| IBIS file stm32f413_f423_wlcsp81.ibs
[IBIS ver] 4.2
[File name] stm32f413_f423_wlcsp81.ibs
[File Rev] 1.1
[Date]  18-05-2020
[Source] Data Created at STMicroelectronics
[Notes]  File originated from ELDO simulations. rev 1.1: removal of the rising/falling waveform I2C
[Disclaimer]  This information is for modeling purpose only and is
   not guaranted. The information is subject to change without
   notice.
[Copyright] Copyright 2020 STMicroelectronics Inc.
|   Component stm32f413_f423_wlcsp81
[Component] stm32f413_f423_wlcsp81
[Manufacturer] STMicroelectronics
[Package]
| variable   typ   min   max
R_pkg   0.0   0.0   0.0
L_pkg   0.0H   0.0H   0.0H
C_pkg   0.0F   0.0F   0.0F
[Pin]  signal_name   model_name   R_pin   L_pin   C_pin
A1 VDD_2_0 POWER
A2 PC10 io8p_arsudq_ft
A3 PA15 io8p_arsudq_ft
A4 PD0 io8p_arsudq_ft
A5 PB3 io8p_arsudq_i2c_ft
A6 PB5 io8p_ar3wsudq_ft
A7 BOOT0 vpp_test_hv
A8 VSS_3 GND
A9 VDD_3 POWER
B1 VSS_2_0 POWER
B2 PA14 io8p_arsudq_ft
B3 PA12 io8usb_lsfs_otg_ft
B4 PC12 io8p_arsudq_ft
B5 PB4 io8p_arsudq_i2cin_ft
B6 PB6 io8p_arsudq_i2cin_ft
B7 PB7 io8p_arsudq_i2cin_ft
B8 VSS GND
B9 VBAT POWER
C1 VCAP2_0 POWER
C2 PA13 io8p_arsudq_ft
C3 PA11 io8usb_lsfs_otg_ft
C4 PC11 io8p_arsudq_ft
C5 PD2 io8p_arsudq_ft
C6 PB8 io8p_arsudq_i2cin_ft
C7 PC1 io8p_arwsudq_ft_v33
C8 PC13-ANTI_TAMP io8p_arwsudq_ft_v33
C9 PC14-OSC32_IN io8p_arwsudq_ft
D1 PA10 io8usb_id_otg_ft
D2 PA9 io8usb_vbus_otg_ft
D3 PA8 io8p_arsudq_i2cin_ft
D4 PC7 io8p_arsudq_i2c_ft
D5 PC6 io8p_arsudq_i2c_ft
D6 PB9 io8p_arsudq_i2cin_ft
D7 PC2 io8p_arwsudq_ft
D8 VSS_5 GND
D9 PC15-OSC32_OUT io8p_arsudq_ft
E1 PC8 io8p_arsudq_ft
E2 PC9 io8p_arsudq_i2cin_ft
E3 PB14 io8p_arsudq_i2c_ft
E4 PB0 io8p_ar3wsudq_ft
E5 PA4 io8p_ar3wsudq_ft
E6 PA3 io8p_arwsudq_ft
E7 PC3 io8p_arwsudq_ft
E8 VDD_5 POWER
E9 PH0-OSC_IN io8p_arsudq_ft
F1 VDD_2_USB33 POWER
F2 PD9 io8p_arsudq_ft
F3 PB12 io8p_arsudq_ft
F4 PE13 io8p_arsudq_ft
F5 PA6 io8p_ar3wsudq_ft
F6 VSS GND
F7 VDDA POWER
F8 PC0 io8p_arwsudq_ft_v33
F9 PH1-OSC_OUT io8p_arsudq_ft
G1 PD10 io8p_arsudq_ft
G2 PB13 io8p_arsudq_ft
G3 PE14 io8p_arsudq_ft
G4 PE10 io8p_arsudq_ft
G5 PB1 io8p_ar3wsudq_ft
G6 PA5 io8p_ar3wsudq_ft
G7 PA0-WKUP io8p_arwsudq_ft_v33
G8 VREF+ POWER
G9 NRST ioreset_ft_v33
H1 PB15 io8p_arsudq_i2c_ft
H2 VCAP1_0 POWER
H3 PB10 io8p_arsudq_i2c_ft
H4 PE11 io8p_arsudq_ft
H5 PB2 io8p_arwsudq_ft
H6 PC4 io8p_arwsudq_ft
H7 VSS_4 GND
H8 PA1 io8p_arwsudq_ft
H9 VSSA GND
J1 VDD_1_0 POWER
J2 VSS_1_0 GND
J3 PE15 io8p_ar3wsudq_ft
J4 PE12 io8p_arsudq_ft
J5 PE9 io8p_arsudq_ft
J6 PC5 io8p_arwsudq_ft
J7 PA7 io8p_arwsudq_ft
J8 VDD_4 POWER
J9 PA2 io8p_arwsudq_ft
[Model Selector] io8p_ar3wsudq_ft
io8p00_ar3wsudq_ft_pd_lv  "SPEED00 1P8V, PD=40kOhm"
io8p00_ar3wsudq_ft_pu_lv  "SPEED00 1P8V, PU=40kOhm"
io8p00_ar3wsudq_ft_lv  "SPEED00 1P8V"
io8p01_ar3wsudq_ft_pd_lv  "SPEED01 1P8V, PD=40kOhm"
io8p01_ar3wsudq_ft_pu_lv  "SPEED01 1P8V, PU=40kOhm"
io8p01_ar3wsudq_ft_lv  "SPEED01 1P8V"
io8p10_ar3wsudq_ft_pd_lv  "SPEED10 1P8V, PD=40kOhm"
io8p10_ar3wsudq_ft_pu_lv  "SPEED10 1P8V, PU=40kOhm"
io8p10_ar3wsudq_ft_lv  "SPEED10 1P8V"
io8p11_ar3wsudq_ft_pd_lv  "SPEED11 1P8V, PD=40kOhm"
io8p11_ar3wsudq_ft_pu_lv  "SPEED11 1P8V, PU=40kOhm"
io8p11_ar3wsudq_ft_lv  "SPEED11 1P8V"
io8p00_ar3wsudq_ft_pd  "SPEED00, PD=40kOhm"
io8p00_ar3wsudq_ft_pu  "SPEED00, PU=40kOhm"
io8p00_ar3wsudq_ft  "SPEED00"
io8p01_ar3wsudq_ft_pd  "SPEED01, PD=40kOhm"
io8p01_ar3wsudq_ft_pu  "SPEED01, PU=40kOhm"
io8p01_ar3wsudq_ft  "SPEED01"
io8p10_ar3wsudq_ft_pd  "SPEED10, PD=40kOhm"
io8p10_ar3wsudq_ft_pu  "SPEED10, PU=40kOhm"
io8p10_ar3wsudq_ft  "SPEED10"
io8p11_ar3wsudq_ft_pd  "SPEED11, PD=40kOhm"
io8p11_ar3wsudq_ft_pu  "SPEED11, PU=40kOhm"
io8p11_ar3wsudq_ft  "SPEED11"
[Model Selector] io8p_arsudq_ft
io8p00_arsudq_ft_pd_lv  "SPEED00 1P8V, PD=40kOhm"
io8p00_arsudq_ft_pu_lv  "SPEED00 1P8V, PU=40kOhm"
io8p00_arsudq_ft_lv  "SPEED00 1P8V"
io8p01_arsudq_ft_pd_lv  "SPEED01 1P8V, PD=40kOhm"
io8p01_arsudq_ft_pu_lv  "SPEED01 1P8V, PU=40kOhm"
io8p01_arsudq_ft_lv  "SPEED01 1P8V"
io8p10_arsudq_ft_pd_lv  "SPEED10 1P8V, PD=40kOhm"
io8p10_arsudq_ft_pu_lv  "SPEED10 1P8V, PU=40kOhm"
io8p10_arsudq_ft_lv  "SPEED10 1P8V"
io8p11_arsudq_ft_pd_lv  "SPEED11 1P8V, PD=40kOhm"
io8p11_arsudq_ft_pu_lv  "SPEED11 1P8V, PU=40kOhm"
io8p11_arsudq_ft_lv  "SPEED11 1P8V"
io8p00_arsudq_ft_pd  "SPEED00, PD=40kOhm"
io8p00_arsudq_ft_pu  "SPEED00, PU=40kOhm"
io8p00_arsudq_ft  "SPEED00"
io8p01_arsudq_ft_pd  "SPEED01, PD=40kOhm"
io8p01_arsudq_ft_pu  "SPEED01, PU=40kOhm"
io8p01_arsudq_ft  "SPEED01"
io8p10_arsudq_ft_pd  "SPEED10, PD=40kOhm"
io8p10_arsudq_ft_pu  "SPEED10, PU=40kOhm"
io8p10_arsudq_ft  "SPEED10"
io8p11_arsudq_ft_pd  "SPEED11, PD=40kOhm"
io8p11_arsudq_ft_pu  "SPEED11, PU=40kOhm"
io8p11_arsudq_ft  "SPEED11"
[Model Selector] io8p_arsudq_i2c_ft
io8prog_1v8_i2c_pd  "5V Tol GPIO 1.8V range i2c functionality with pull down"
io8prog_1v8_i2c_pu  "5V Tol GPIO 1.8V range i2c functionality with pull up"
io8prog_1v8_i2c  "5V Tol GPIO 1.8V range i2c functionality"
io8prog_3v3_i2c_pd  "5V Tol GPIO 3.3V range i2c functionality with pull down"
io8prog_3v3_i2c_pu  "5V Tol GPIO 3.3V range i2c functionality with pull up"
io8prog_3v3_i2c  "5V Tol GPIO 3.3V range i2c functionality"
io8prog_1v8_pd_00  "5V Tol GPIO 1.8V range with pd speed 00"
io8prog_1v8_pu_00  "5V Tol GPIO 1.8V range with pu speed 00"
io8prog_1v8_00  "5V Tol GPIO 1.8V range speed 00"
io8prog_3v3_pd_00  "5V Tol GPIO 3.3V range with pd speed 00"
io8prog_3v3_pu_00  "5V Tol GPIO 3.3V range with pu speed 00"
io8prog_3v3_00  "5V Tol GPIO 3.3V range speed 00"
io8prog_1v8_pd_01  "5V Tol GPIO 1.8V range with pd speed 01"
io8prog_1v8_pu_01  "5V Tol GPIO 1.8V range with pu speed 01"
io8prog_1v8_01  "5V Tol GPIO 1.8V range speed 01"
io8prog_3v3_pd_01  "5V Tol GPIO 3.3V range with pd speed 01"
io8prog_3v3_pu_01  "5V Tol GPIO 3.3V range with pu speed 01"
io8prog_3v3_01  "5V Tol GPIO 3.3V range speed 01"
io8prog_1v8_pd_10  "5V Tol GPIO 1.8V range with pd speed 10"
io8prog_1v8_pu_10  "5V Tol GPIO 1.8V range with pu speed 10"
io8prog_1v8_10  "5V Tol GPIO 1.8V range speed 10"
io8prog_3v3_pd_10  "5V Tol GPIO 3.3V range with pd speed 10"
io8prog_3v3_pu_10  "5V Tol GPIO 3.3V range with pu speed 10"
io8prog_3v3_10  "5V Tol GPIO 3.3V range speed 10"
io8prog_1v8_pd_11  "5V Tol GPIO 1.8V range with pd speed 11"
io8prog_1v8_pu_11  "5V Tol GPIO 1.8V range with pu speed 11"
io8prog_1v8_11  "5V Tol GPIO 1.8V range speed 11"
io8prog_3v3_pd_11  "5V Tol GPIO 3.3V range with pd speed 11"
io8prog_3v3_pu_11  "5V Tol GPIO 3.3V range with pu speed 11"
io8prog_3v3_11  "5V Tol GPIO 3.3V range speed 11"
[Model Selector] io8p_arsudq_i2cin_ft
io8p00_arsudq_i2cin_ft_pd_lv  "SPEED00 1P8V, PD=40kOhm"
io8p00_arsudq_i2cin_ft_pu_lv  "SPEED00 1P8V, PU=40kOhm"
io8p00_arsudq_i2cin_ft_lv  "SPEED00 1P8V"
io8p01_arsudq_i2cin_ft_pd_lv  "SPEED01 1P8V, PD=40kOhm"
io8p01_arsudq_i2cin_ft_pu_lv  "SPEED01 1P8V, PU=40kOhm"
io8p01_arsudq_i2cin_ft_lv  "SPEED01 1P8V"
io8p10_arsudq_i2cin_ft_pd_lv  "SPEED10 1P8V, PD=40kOhm"
io8p10_arsudq_i2cin_ft_pu_lv  "SPEED10 1P8V, PU=40kOhm"
io8p10_arsudq_i2cin_ft_lv  "SPEED10 1P8V"
io8p11_arsudq_i2cin_ft_pd_lv  "SPEED11 1P8V, PD=40kOhm"
io8p11_arsudq_i2cin_ft_pu_lv  "SPEED11 1P8V, PU=40kOhm"
io8p11_arsudq_i2cin_ft_lv  "SPEED11 1P8V"
io8p00_arsudq_i2cin_ft_pd  "SPEED00, PD=40kOhm"
io8p00_arsudq_i2cin_ft_pu  "SPEED00, PU=40kOhm"
io8p00_arsudq_i2cin_ft  "SPEED00"
io8p01_arsudq_i2cin_ft_pd  "SPEED01, PD=40kOhm"
io8p01_arsudq_i2cin_ft_pu  "SPEED01, PU=40kOhm"
io8p01_arsudq_i2cin_ft  "SPEED01"
io8p10_arsudq_i2cin_ft_pd  "SPEED10, PD=40kOhm"
io8p10_arsudq_i2cin_ft_pu  "SPEED10, PU=40kOhm"
io8p10_arsudq_i2cin_ft  "SPEED10"
io8p11_arsudq_i2cin_ft_pd  "SPEED11, PD=40kOhm"
io8p11_arsudq_i2cin_ft_pu  "SPEED11, PU=40kOhm"
io8p11_arsudq_i2cin_ft  "SPEED11"
[Model Selector] io8p_arwsudq_ft
io8p00_arwsudq_ft_pd_lv  "SPEED00 1P8V, PD=40kOhm"
io8p00_arwsudq_ft_pu_lv  "SPEED00 1P8V, PU=40kOhm"
io8p00_arwsudq_ft_lv  "SPEED00 1P8V"
io8p01_arwsudq_ft_pd_lv  "SPEED01 1P8V, PD=40kOhm"
io8p01_arwsudq_ft_pu_lv  "SPEED01 1P8V, PU=40kOhm"
io8p01_arwsudq_ft_lv  "SPEED01 1P8V"
io8p10_arwsudq_ft_pd_lv  "SPEED10 1P8V, PD=40kOhm"
io8p10_arwsudq_ft_pu_lv  "SPEED10 1P8V, PU=40kOhm"
io8p10_arwsudq_ft_lv  "SPEED10 1P8V"
io8p11_arwsudq_ft_pd_lv  "SPEED11 1P8V, PD=40kOhm"
io8p11_arwsudq_ft_pu_lv  "SPEED11 1P8V, PU=40kOhm"
io8p11_arwsudq_ft_lv  "SPEED11 1P8V"
io8p00_arwsudq_ft_pd  "SPEED00, PD=40kOhm"
io8p00_arwsudq_ft_pu  "SPEED00, PU=40kOhm"
io8p00_arwsudq_ft  "SPEED00"
io8p01_arwsudq_ft_pd  "SPEED01, PD=40kOhm"
io8p01_arwsudq_ft_pu  "SPEED01, PU=40kOhm"
io8p01_arwsudq_ft  "SPEED01"
io8p10_arwsudq_ft_pd  "SPEED10, PD=40kOhm"
io8p10_arwsudq_ft_pu  "SPEED10, PU=40kOhm"
io8p10_arwsudq_ft  "SPEED10"
io8p11_arwsudq_ft_pd  "SPEED11, PD=40kOhm"
io8p11_arwsudq_ft_pu  "SPEED11, PU=40kOhm"
io8p11_arwsudq_ft  "SPEED11"
[Model Selector] io8p_arwsudq_ft_v33
io8p00_arwsudq_ft_v33_pd_lv  "SPEED00 1P8V, PD=40kOhm"
io8p00_arwsudq_ft_v33_pu_lv  "SPEED00 1P8V, PU=40kOhm"
io8p00_arwsudq_ft_v33_lv  "SPEED00 1P8V"
io8p01_arwsudq_ft_v33_pd_lv  "SPEED01 1P8V, PD=40kOhm"
io8p01_arwsudq_ft_v33_pu_lv  "SPEED01 1P8V, PU=40kOhm"
io8p01_arwsudq_ft_v33_lv  "SPEED01 1P8V"
io8p10_arwsudq_ft_v33_pd_lv  "SPEED10 1P8V, PD=40kOhm"
io8p10_arwsudq_ft_v33_pu_lv  "SPEED10 1P8V, PU=40kOhm"
io8p10_arwsudq_ft_v33_lv  "SPEED10 1P8V"
io8p11_arwsudq_ft_v33_pd_lv  "SPEED11 1P8V, PD=40kOhm"
io8p11_arwsudq_ft_v33_pu_lv  "SPEED11 1P8V, PU=40kOhm"
io8p11_arwsudq_ft_v33_lv  "SPEED11 1P8V"
io8p00_arwsudq_ft_v33_pd  "SPEED00, PD=40kOhm"
io8p00_arwsudq_ft_v33_pu  "SPEED00, PU=40kOhm"
io8p00_arwsudq_ft_v33  "SPEED00"
io8p01_arwsudq_ft_v33_pd  "SPEED01, PD=40kOhm"
io8p01_arwsudq_ft_v33_pu  "SPEED01, PU=40kOhm"
io8p01_arwsudq_ft_v33  "SPEED01"
io8p10_arwsudq_ft_v33_pd  "SPEED10, PD=40kOhm"
io8p10_arwsudq_ft_v33_pu  "SPEED10, PU=40kOhm"
io8p10_arwsudq_ft_v33  "SPEED10"
io8p11_arwsudq_ft_v33_pd  "SPEED11, PD=40kOhm"
io8p11_arwsudq_ft_v33_pu  "SPEED11, PU=40kOhm"
io8p11_arwsudq_ft_v33  "SPEED11"
[Model Selector] io8usb_id_otg_ft
io8p00_id_otg_ft_pd_lv  "SPEED00 1P8V, PD=14kOhm"
io8p00_id_otg_ft_pu_lv  "SPEED00 1P8V, PU=14kOhm"
io8p00_id_otg_ft_lv  "SPEED00 1P8V"
io8p01_id_otg_ft_pd_lv  "SPEED01 1P8V, PD=14kOhm"
io8p01_id_otg_ft_pu_lv  "SPEED01 1P8V, PU=14kOhm"
io8p01_id_otg_ft_lv  "SPEED01 1P8V"
io8p10_id_otg_ft_pd_lv  "SPEED10 1P8V, PD=14kOhm"
io8p10_id_otg_ft_pu_lv  "SPEED10 1P8V, PU=14kOhm"
io8p10_id_otg_ft_lv  "SPEED10 1P8V"
io8p11_id_otg_ft_pd_lv  "SPEED11 1P8V, PD=14kOhm"
io8p11_id_otg_ft_pu_lv  "SPEED11 1P8V, PU=14kOhm"
io8p11_id_otg_ft_lv  "SPEED11 1P8V"
io8p00_id_otg_ft_pd  "SPEED00, PD=14kOhm"
io8p00_id_otg_ft_pu  "SPEED00, PU=14kOhm"
io8p00_id_otg_ft  "SPEED00"
io8p01_id_otg_ft_pd  "SPEED01, PD=14kOhm"
io8p01_id_otg_ft_pu  "SPEED01, PU=14kOhm"
io8p01_id_otg_ft  "SPEED01"
io8p10_id_otg_ft_pd  "SPEED10, PD=14kOhm"
io8p10_id_otg_ft_pu  "SPEED10, PU=14kOhm"
io8p10_id_otg_ft  "SPEED10"
io8p11_id_otg_ft_pd  "SPEED11, PD=14kOhm"
io8p11_id_otg_ft_pu  "SPEED11, PU=14kOhm"
io8p11_id_otg_ft  "SPEED11"
[Model Selector] io8usb_lsfs_otg_ft
io8usb_ls_otg_ft_dpdn_pd  "LS USB DP/DN IO + PD=20kOhm"
io8usb_ls_otg_ft_dpdn_pupu2  "LS USB DP/DN IO + PU/PU2=2.2kOhm"
io8usb_ls_otg_ft_dpdn_pu2  "LS USB DP/DN IO + PU2=1.2kOhm"
io8usb_ls_otg_ft_dpdn_pu  "LS USB DP/DN IO + PU=1.2kOhm"
io8usb_ls_otg_ft_dpdn  "LS USB DP/DN IO"
io8usb_fs_otg_ft_dpdn_pd  "HS USB DP/DN IO + PD=20kOhm"
io8usb_fs_otg_ft_dpdn_pupu2  "HS USB DP/DN IO + PU/PU2=2.2kOhm"
io8usb_fs_otg_ft_dpdn_pu2  "HS USB DP/DN IO + PU2=1.2kOhm"
io8usb_fs_otg_ft_dpdn_pu  "HS USB DP/DN IO + PU=1.2kOhm"
io8usb_fs_otg_ft_dpdn  "HS USB DP/DN IO"
io8p00_lsfs_otg_ft_pd_lv  "SPEED00 1P8V, PD=40kOhm"
io8p00_lsfs_otg_ft_pu_lv  "SPEED00 1P8V, PU=40kOhm"
io8p00_lsfs_otg_ft_lv  "SPEED00 1P8V"
io8p01_lsfs_otg_ft_pd_lv  "SPEED01 1P8V, PD=40kOhm"
io8p01_lsfs_otg_ft_pu_lv  "SPEED01 1P8V, PU=40kOhm"
io8p01_lsfs_otg_ft_lv  "SPEED01 1P8V"
io8p10_lsfs_otg_ft_pd_lv  "SPEED10 1P8V, PD=40kOhm"
io8p10_lsfs_otg_ft_pu_lv  "SPEED10 1P8V, PU=40kOhm"
io8p10_lsfs_otg_ft_lv  "SPEED10 1P8V"
io8p11_lsfs_otg_ft_pd_lv  "SPEED11 1P8V, PD=40kOhm"
io8p11_lsfs_otg_ft_pu_lv  "SPEED11 1P8V, PU=40kOhm"
io8p11_lsfs_otg_ft_lv  "SPEED11 1P8V"
io8p00_lsfs_otg_ft_pd  "SPEED00, PD=40kOhm"
io8p00_lsfs_otg_ft_pu  "SPEED00, PU=40kOhm"
io8p00_lsfs_otg_ft  "SPEED00"
io8p01_lsfs_otg_ft_pd  "SPEED01, PD=40kOhm"
io8p01_lsfs_otg_ft_pu  "SPEED01, PU=40kOhm"
io8p01_lsfs_otg_ft  "SPEED01"
io8p10_lsfs_otg_ft_pd  "SPEED10, PD=40kOhm"
io8p10_lsfs_otg_ft_pu  "SPEED10, PU=40kOhm"
io8p10_lsfs_otg_ft  "SPEED10"
io8p11_lsfs_otg_ft_pd  "SPEED11, PD=40kOhm"
io8p11_lsfs_otg_ft_pu  "SPEED11, PU=40kOhm"
io8p11_lsfs_otg_ft  "SPEED11"
[Model Selector] io8usb_vbus_otg_ft
io8psenb_vbus_otg_ft  "VBUS PULSE, SENSE VB"
io8psenab_vbus_otg_ft  "VBUS PULSE, SENSE VA and VB"
io8psena_vbus_otg_ft  "VBUS PULSE, SENSE VA"
io8psen_vbus_otg_ft  "VBUS PULSE"
io8p00_vbus_otg_ft_pd_lv  "SPEED00 1P8V, PD=40kOhm"
io8p00_vbus_otg_ft_pu_lv  "SPEED00 1P8V, PU=40kOhm"
io8p00_vbus_otg_ft_lv  "SPEED00 1P8V"
io8p01_vbus_otg_ft_pd_lv  "SPEED01 1P8V, PD=40kOhm"
io8p01_vbus_otg_ft_pu_lv  "SPEED01 1P8V, PU=40kOhm"
io8p01_vbus_otg_ft_lv  "SPEED01 1P8V"
io8p10_vbus_otg_ft_pd_lv  "SPEED10 1P8V, PD=40kOhm"
io8p10_vbus_otg_ft_pu_lv  "SPEED10 1P8V, PU=40kOhm"
io8p10_vbus_otg_ft_lv  "SPEED10 1P8V"
io8p11_vbus_otg_ft_pd_lv  "SPEED11 1P8V, PD=40kOhm"
io8p11_vbus_otg_ft_pu_lv  "SPEED11 1P8V, PU=40kOhm"
io8p11_vbus_otg_ft_lv  "SPEED11 1P8V"
io8p00_vbus_otg_ft_pd  "SPEED00, PD=40kOhm"
io8p00_vbus_otg_ft_pu  "SPEED00, PU=40kOhm"
io8p00_vbus_otg_ft  "SPEED00"
io8p01_vbus_otg_ft_pd  "SPEED01, PD=40kOhm"
io8p01_vbus_otg_ft_pu  "SPEED01, PU=40kOhm"
io8p01_vbus_otg_ft  "SPEED01"
io8p10_vbus_otg_ft_pd  "SPEED10, PD=40kOhm"
io8p10_vbus_otg_ft_pu  "SPEED10, PU=40kOhm"
io8p10_vbus_otg_ft  "SPEED10"
io8p11_vbus_otg_ft_pd  "SPEED11, PD=40kOhm"
io8p11_vbus_otg_ft_pu  "SPEED11, PU=40kOhm"
io8p11_vbus_otg_ft  "SPEED11"
[Model Selector] ioreset_ft_v33
ioreset_ft_v33_pu_lv  "IORESET 1P8V + PU=40kOhm"
ioreset_ft_v33_nopu_lv  "IORESET 1P8V"
ioreset_ft_v33_pu  "IORESET + PU=40kOhm"
ioreset_ft_v33_nopu  "IORESET"
[Model Selector] vpp_test_hv
vpp_test_hv_2p4  "Input Buffer 1P8V"
vpp_test_hv_3p3  "Input Buffer"
| Models and submodels in the file (242): io8p00_ar3wsudq_ft_pd_lv (I/O), io8p00_ar3wsudq_ft_pu_lv (I/O), io8p00_ar3wsudq_ft_lv (I/O), io8p01_ar3wsudq_ft_pd_lv (I/O), io8p01_ar3wsudq_ft_pu_lv (I/O), io8p01_ar3wsudq_ft_lv (I/O), io8p10_ar3wsudq_ft_pd_lv (I/O), io8p10_ar3wsudq_ft_pu_lv (I/O), io8p10_ar3wsudq_ft_lv (I/O), io8p11_ar3wsudq_ft_pd_lv (I/O), io8p11_ar3wsudq_ft_pu_lv (I/O), io8p11_ar3wsudq_ft_lv (I/O), io8p00_ar3wsudq_ft_pd (I/O), io8p00_ar3wsudq_ft_pu (I/O), io8p00_ar3wsudq_ft (I/O), io8p01_ar3wsudq_ft_pd (I/O), io8p01_ar3wsudq_ft_pu (I/O), io8p01_ar3wsudq_ft (I/O), io8p10_ar3wsudq_ft_pd (I/O), io8p10_ar3wsudq_ft_pu (I/O), io8p10_ar3wsudq_ft (I/O), io8p11_ar3wsudq_ft_pd (I/O), io8p11_ar3wsudq_ft_pu (I/O), io8p11_ar3wsudq_ft (I/O), io8p00_arsudq_ft_pd_lv (I/O), io8p00_arsudq_ft_pu_lv (I/O), io8p00_arsudq_ft_lv (I/O), io8p01_arsudq_ft_pd_lv (I/O), io8p01_arsudq_ft_pu_lv (I/O), io8p01_arsudq_ft_lv (I/O), io8p10_arsudq_ft_pd_lv (I/O), io8p10_arsudq_ft_pu_lv (I/O), io8p10_arsudq_ft_lv (I/O), io8p11_arsudq_ft_pd_lv (I/O), io8p11_arsudq_ft_pu_lv (I/O), io8p11_arsudq_ft_lv (I/O), io8p00_arsudq_ft_pd (I/O), io8p00_arsudq_ft_pu (I/O), io8p00_arsudq_ft (I/O), io8p01_arsudq_ft_pd (I/O), io8p01_arsudq_ft_pu (I/O), io8p01_arsudq_ft (I/O), io8p10_arsudq_ft_pd (I/O), io8p10_arsudq_ft_pu (I/O), io8p10_arsudq_ft (I/O), io8p11_arsudq_ft_pd (I/O), io8p11_arsudq_ft_pu (I/O), io8p11_arsudq_ft (I/O), io8prog_1v8_i2c_pd (I/O), io8prog_1v8_i2c_pu (I/O), io8prog_1v8_i2c (I/O), io8prog_3v3_i2c_pd (I/O), io8prog_3v3_i2c_pu (I/O), io8prog_3v3_i2c (I/O), io8prog_1v8_pd_00 (I/O), io8prog_1v8_pu_00 (I/O), io8prog_1v8_00 (I/O), io8prog_3v3_pd_00 (I/O), io8prog_3v3_pu_00 (I/O), io8prog_3v3_00 (I/O), io8prog_1v8_pd_01 (I/O), io8prog_1v8_pu_01 (I/O), io8prog_1v8_01 (I/O), io8prog_3v3_pd_01 (I/O), io8prog_3v3_pu_01 (I/O), io8prog_3v3_01 (I/O), io8prog_1v8_pd_10 (I/O), io8prog_1v8_pu_10 (I/O), io8prog_1v8_10 (I/O), io8prog_3v3_pd_10 (I/O), io8prog_3v3_pu_10 (I/O), io8prog_3v3_10 (I/O), io8prog_1v8_pd_11 (I/O), io8prog_1v8_pu_11 (I/O), io8prog_1v8_11 (I/O), io8prog_3v3_pd_11 (I/O), io8prog_3v3_pu_11 (I/O), io8prog_3v3_11 (I/O), io8p00_arsudq_i2cin_ft_pd_lv (I/O), io8p00_arsudq_i2cin_ft_pu_lv (I/O)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
